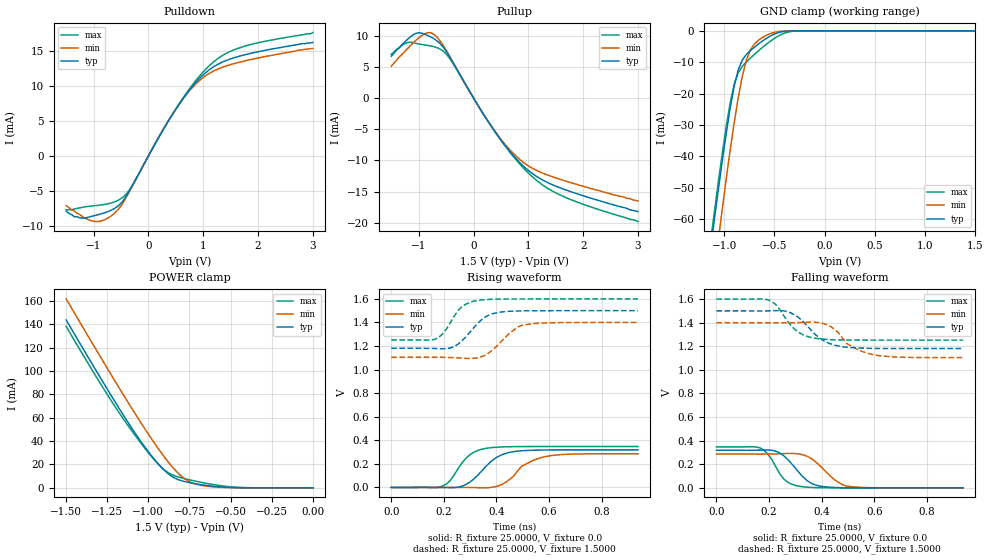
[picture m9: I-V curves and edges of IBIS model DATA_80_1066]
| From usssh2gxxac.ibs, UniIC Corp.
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|   Model DATA_80_1066
[Model]  DATA_80_1066
Model_type I/O
Polarity   Non-Inverting
Enable   Active-High
Vinl =   0.60000000V
Vinh =   0.90000000V
Vmeas =   0.750000000V
Rref =   25.00000000
Vref =   0.75000000V
C_comp   1.6160pF   1.5990pF   1.6430pF
[Temperature Range]   25.0000   95.0000   0.0
[Voltage Range]   1.5000V   1.4000V   1.6000V
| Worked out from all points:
|   slope of the pulldown table from 0 to 0.225 V, typ, clamps not added: 70.9 ohm
|   slope of the pullup table from 0 to 0.225 V, typ, clamps not added: 70 ohm
|   GND clamp passes 1 mA (typ) near -0.50 V on its own axis
|   POWER clamp passes 1 mA (typ) near -0.58 V on its own axis
|   rising waveform, R_fixture 25.0000, V_fixture 0.0: 20-80 % time 91.5ps typ, 95.7ps min, 71.4ps max; typ from 0 V to 0.319 V
|   rising waveform, R_fixture 25.0000, V_fixture 1.5000: 20-80 % time 82.5ps typ, 85.9ps min, 65.7ps max; typ from 1.18 V to 1.5 V
|   falling waveform, R_fixture 25.0000, V_fixture 0.0: 20-80 % time 79.2ps typ, 84.7ps min, 61.1ps max; typ from 0.319 V to 0 V
|   falling waveform, R_fixture 25.0000, V_fixture 1.5000: 20-80 % time 93.8ps typ, 95.3ps min, 77ps max; typ from 1.5 V to 1.18 V
[Pulldown]
|Voltage   I(typ)   I(min)   I(max)
-1.5V     -7.9mA     -7.1mA     -7.7mA
-1.25V    -8.86mA    -8.4mA     -7.43mA
-1V       -8.57mA    -9.35mA    -7.13mA
-800mV    -8.135mA   -9.13mA    -6.94mA
-600mV    -7.422mA   -8.068mA   -6.512mA
-350mV    -5.045mA   -5.146mA   -4.893mA
200mV     2.832mA    2.856mA    2.829mA
550mV     7.292mA    7.282mA    7.356mA
850mV     10.41mA    10.22mA    10.67mA
1.15V     12.59mA    12.03mA    13.23mA
1.7V      14.4mA     13.53mA    15.61mA
3V        16.3mA     15.4mA     17.7mA
[Pullup]
|Voltage   I(typ)   I(min)   I(max)
-1.5V     6.7mA      5.1mA      7mA
-1.25V    9mA        7.5mA      8.72mA
-1.05V    10.35mA    9.26mA     8.76mA
-900mV    10.25mA    10.25mA    8.51mA
-750mV    9.639mA    10.35mA    8.28mA
-600mV    8.621mA    9.028mA    7.779mA
-450mV    6.804mA    6.923mA    6.517mA
350mV     -4.882mA   -4.81mA    -4.873mA
900mV     -10.83mA   -10.26mA   -11.12mA
1.2V      -12.84mA   -11.81mA   -13.54mA
1.55V     -14.29mA   -12.95mA   -15.42mA
3V        -18.2mA    -16.5mA    -19.8mA
[GND_clamp]
|Voltage   I(typ)   I(min)   I(max)
-1.5V     -169mA     -189.1mA   -163.8mA
-1.14V    -70.71mA   -88.3mA    -68.32mA
-1.1V     -60.74mA   -77.66mA   -58.33mA
-1.06V    -51.03mA   -67.22mA   -48.61mA
-1.02V    -41.65mA   -57.06mA   -39.27mA
-940mV    -24.55mA   -37.9mA    -22.88mA
-860mV    -12.39mA   -21.26mA   -13.32mA
-780mV    -7.577mA   -9.433mA   -9.942mA
-740mV    -6.329mA   -6.125mA   -8.71mA
-620mV    -3.273mA   -2.113mA   -5.305mA
-300mV    -11.81uA   -4.878uA   -91.71uA
1.5V      4.577nA    23.6nA     33.33nA
[POWER_clamp]
|Voltage   I(typ)   I(min)   I(max)
-1.5V     143.7mA    161.7mA    138.1mA
-1.22V    77.56mA    95.29mA    73.32mA
-1.12V    55.19mA    72.34mA    52.54mA
-1.02V    34.59mA    50.23mA    33.56mA
-960mV    23.77mA    37.63mA    23.28mA
-900mV    14.66mA    25.9mA     15mA
-840mV    8.415mA    15.63mA    10.28mA
-780mV    5.408mA    7.848mA    7.861mA
-700mV    3.206mA    2.693mA    5.332mA
-600mV    1.29mA     794.5uA    2.681mA
-420mV    69.47uA    44.47uA    238.7uA
0V        4.577nA    6.249nA    39.08nA
[Ramp]
| variable   typ   min   max
dV/dt_r  0.1912/91.4560p   0.1717/0.1057n   0.2083/71.3681p
dV/dt_f  0.1914/93.7667p   0.1776/0.1053n   0.2088/77.0400p
R_load = 25.0000
[Rising Waveform]
R_fixture= 25.0000
V_fixture= 0.0
V_fixture_min= 0.0
V_fixture_max= 0.0
|time   V(typ)   V(min)   V(max)
0s        0V         0V         0V
195ps     -109.1uV   130.4uV    11.92mV
225ps     -2.146mV   295.3uV    60.83mV
285ps     25.97mV    46.45uV    250.4mV
360ps     178.9mV    -3.571mV   331.6mV
435ps     288.6mV    43.53mV    344.6mV
495ps     311.1mV    178.3mV    346.6mV
575ps     317.3mV    256.1mV    347.1mV
680ps     318.5mV    282.3mV    347.2mV
938ps     318.6mV    286.1mV    347.2mV
[Rising Waveform]
R_fixture= 25.0000
V_fixture= 1.5000
V_fixture_min= 1.4000
V_fixture_max= 1.6000
|time   V(typ)   V(min)   V(max)
0s        1.181V     1.104V     1.252V
165ps     1.179V     1.104V     1.256V
195ps     1.176V     1.104V     1.303V
240ps     1.196V     1.101V     1.456V
270ps     1.247V     1.097V     1.536V
330ps     1.396V     1.101V     1.587V
390ps     1.477V     1.176V     1.597V
450ps     1.495V     1.308V     1.599V
495ps     1.498V     1.375V     1.599V
938ps     1.5V       1.4V       1.6V
[Falling Waveform]
R_fixture= 25.0000
V_fixture= 0.0
V_fixture_min= 0.0
V_fixture_max= 0.0
|time   V(typ)   V(min)   V(max)
0s        318.6mV    286.1mV    347.2mV
165ps     319.9mV    285.8mV    339.5mV
195ps     320.8mV    286.3mV    287mV
240ps     297.5mV    288.7mV    122.6mV
270ps     242.8mV    291.5mV    49.29mV
315ps     127.1mV    286.6mV    13.32mV
375ps     25.28mV    224.3mV    2.273mV
450ps     2.981mV    67.16mV    253.7uV
495ps     807.6uV    14.55mV    65.4uV
938ps     0V         0V         0V
[Falling Waveform]
R_fixture= 25.0000
V_fixture= 1.5000
V_fixture_min= 1.4000
V_fixture_max= 1.6000
|time   V(typ)   V(min)   V(max)
0s        1.5V       1.4V       1.6V
195ps     1.5V       1.399V     1.594V
225ps     1.502V     1.399V     1.555V
285ps     1.481V     1.4V       1.373V
330ps     1.409V     1.403V     1.297V
375ps     1.302V     1.404V     1.268V
450ps     1.209V     1.342V     1.255V
495ps     1.192V     1.224V     1.253V
590ps     1.182V     1.132V     1.252V
938ps     1.181V     1.104V     1.252V
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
